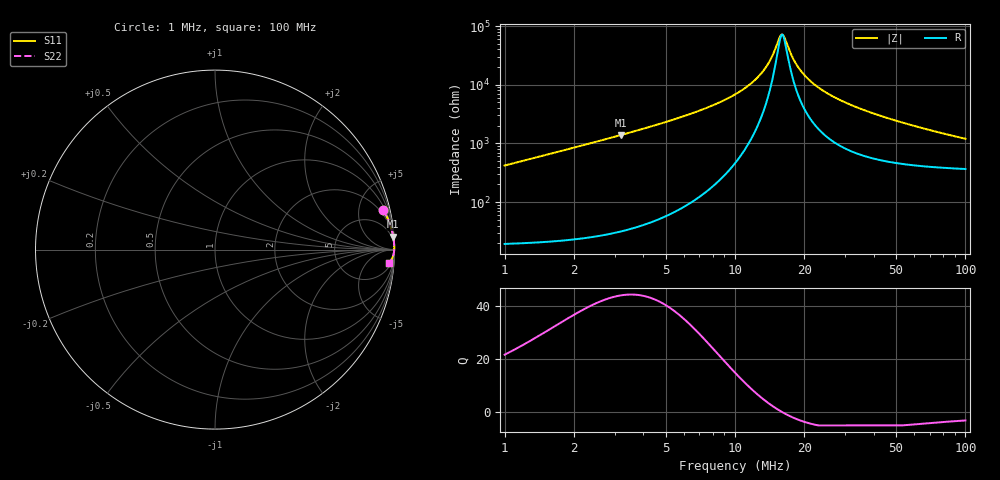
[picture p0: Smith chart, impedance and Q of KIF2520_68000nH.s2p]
!version-2
!date-12.2020
!Series
# MHz S RI R 50
!Freq ReS11 ImS11 ReS21 ImS21 ReS12 ImS12 ReS22 ImS22
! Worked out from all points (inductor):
!   991 points, 1 MHz to 100 MHz, reference 50 ohm
!   read as one part in series: L = 66.4 uH near 1.4 MHz
!   highest Q = 43.6 at 3.2 MHz (marker M1), where L = 69.2 uH
!   self-resonance near 16 MHz
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1  0.9372 0.2205  0.0628 -0.2205  0.0628 -0.2205  0.9372 0.2205
2.1  0.9848 0.11  0.0152 -0.11  0.0152 -0.11  0.9848 0.11
3.2  0.9933 0.0712  0.00674 -0.0712  0.00674 -0.0712  0.9933 0.0712
5.1  0.9972 0.042  0.00283 -0.042  0.00283 -0.042  0.9972 0.042
10.2  0.9988 0.0139  0.00119 -0.0139  0.00119 -0.0139  0.9988 0.0139
12.3  0.9988 0.00799  0.00117 -0.00799  0.00117 -0.00799  0.9988 0.00799
14  0.9988 0.00405  0.00124 -0.00405  0.00124 -0.00405  0.9988 0.00405
15.8  0.9986 0.000449  0.00137 -0.000449  0.00137 -0.000449  0.9986 0.000449
16.1  0.9986 -0.000109  0.0014 0.000109  0.0014 0.000109  0.9986 -0.000109
16.4  0.9986 -0.000657  0.00143 0.000657  0.00143 0.000657  0.9986 -0.000657
17.5  0.9985 -0.00258  0.00154 0.00258  0.00154 0.00258  0.9985 -0.00258
18.4  0.9984 -0.00408  0.00164 0.00408  0.00164 0.00408  0.9984 -0.00408
19.6  0.9982 -0.00597  0.00179 0.00597  0.00179 0.00597  0.9982 -0.00597
21  0.998 -0.00806  0.00199 0.00806  0.00199 0.00806  0.998 -0.00806
22.8  0.9977 -0.0106  0.00227 0.0106  0.00227 0.0106  0.9977 -0.0106
27.5  0.9969 -0.0166  0.00312 0.0166  0.00312 0.0166  0.9969 -0.0166
34  0.9954 -0.024  0.00457 0.024  0.00457 0.024  0.9954 -0.024
41.3  0.9935 -0.0314  0.00654 0.0314  0.00654 0.0314  0.9935 -0.0314
50.5  0.9905 -0.04  0.00947 0.04  0.00947 0.04  0.9905 -0.04
67  0.9843 -0.0535  0.0157 0.0535  0.0157 0.0535  0.9843 -0.0535
83.5  0.9771 -0.0651  0.0229 0.0651  0.0229 0.0651  0.9771 -0.0651
100  0.9694 -0.0749  0.0306 0.0749  0.0306 0.0749  0.9694 -0.0749
